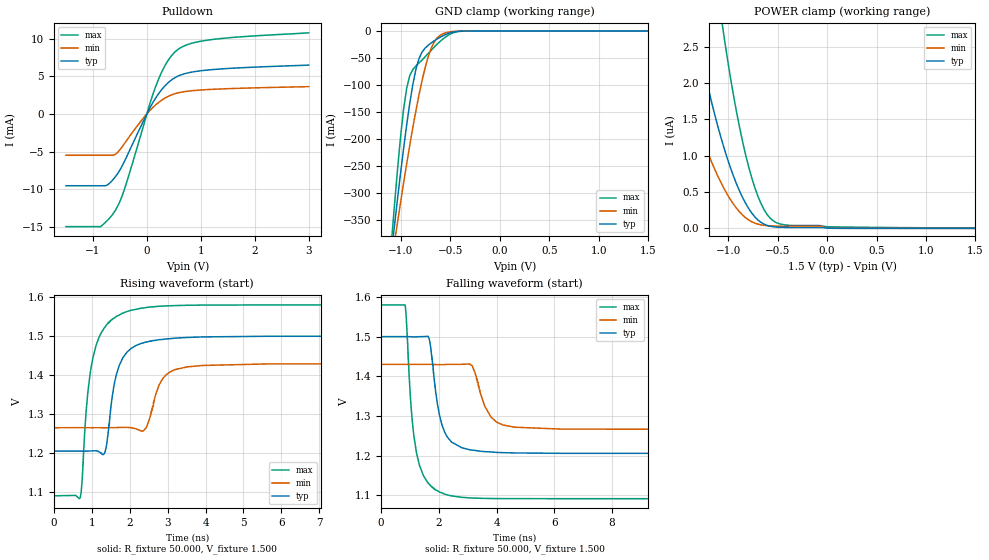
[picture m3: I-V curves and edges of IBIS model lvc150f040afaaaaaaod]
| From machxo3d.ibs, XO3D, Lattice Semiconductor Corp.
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|   Model lvc150f040afaaaaaaod
[Model] lvc150f040afaaaaaaod
Model_type I/O_open_drain
Polarity   Non-Inverting
Enable   Active-Low
Vinl =  0.375V
Vinh =  1.125V
Vmeas =  0.750V
Cref =  0.0F
Rref = 10.00k
Vref = 1.50V
C_comp   4.200pF   3.800pF   7.500pF
[Temperature Range]   25.000   0.105k   -40.000
[Voltage Range]   1.500V   1.430V   1.580V
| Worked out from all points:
|   slope of the pulldown table from 0 to 0.225 V, typ, clamps not added: 81.5 ohm
|   GND clamp passes 1 mA (typ) near -0.44 V on its own axis
|   rising waveform, R_fixture 50.000, V_fixture 1.500: 20-80 % time 357ps typ, 371ps min, 357ps max; typ from 1.21 V to 1.5 V
|   falling waveform, R_fixture 50.000, V_fixture 1.500: 20-80 % time 404ps typ, 495ps min, 361ps max; typ from 1.5 V to 1.21 V
[Pulldown]
|Voltage   I(typ)   I(min)   I(max)
-1.5V     -9.549mA   -5.496mA   -14.98mA
-856mV    -9.549mA   -5.496mA   -14.98mA
-718mV    -9.375mA   -5.496mA   -14.06mA
-580mV    -8.322mA   -5.363mA   -12.78mA
-396mV    -6.022mA   -3.748mA   -9.594mA
64mV      897.8uA    512.6uA    1.542mA
202mV     2.531mA    1.437mA    4.351mA
386mV     4.093mA    2.3mA      7.031mA
570mV     5.004mA    2.786mA    8.534mA
800mV     5.518mA    3.061mA    9.331mA
1.214V    5.895mA    3.272mA    9.897mA
3V        6.493mA    3.63mA     10.79mA
[GND_clamp]
|Voltage   I(typ)   I(min)   I(max)
-1.5V     -1.124A    -960.6mA   -1.411A
-1.097V   -411.6mA   -430.5mA   -392.9mA
-1.066V   -360.7mA   -392.1mA   -323mA
-1.035V   -311mA     -354.2mA   -256.8mA
-973mV    -216.9mA   -280.8mA   -144.3mA
-942mV    -173.5mA   -245.5mA   -105.7mA
-849mV    -71.07mA   -147.7mA   -64.62mA
-787mV    -39.18mA   -92.07mA   -53.7mA
-725mV    -26.42mA   -48.02mA   -41.6mA
-601mV    -11.16mA   -7.547mA   -18.74mA
-384mV    -237.5uA   -103.4uA   -356uA
1.5V      0A         0A         0A
[POWER_clamp]
|Voltage   I(typ)   I(min)   I(max)
-1.5V     4.017uA    2.297uA    8.486uA
-1.321V   2.676uA    1.475uA    5.815uA
-1.166V   1.719uA    902.9nA    3.892uA
-1.073V   1.242uA    625.4nA    2.92uA
-1.042V   1.099uA    544.2nA    2.626uA
-949mV    723.1nA    335.9nA    1.84uA
-856mV    425.6nA    184nA      1.196uA
-763mV    211.1nA    90.94nA    695.6nA
-670mV    83.03nA    48.42nA    343.1nA
-577mV    29.38nA    34.62nA    141nA
-422mV    12.83nA    29.5nA     47.28nA
1.5V      0A         0A         4.136nA
[Ramp]
| variable   typ   min   max
dV/dt_r   0.177/0.358n   98.704m/0.378n   0.293/0.357n
dV/dt_f   0.177/0.405n   98.705m/0.501n   0.293/0.354n
R_load = 50.000
[Rising Waveform]
R_fixture= 50.000
V_fixture= 1.500
V_fixture_min= 1.430
V_fixture_max= 1.580
|time   V(typ)   V(min)   V(max)
0s        1.205V     1.265V     1.091V
697ps     1.206V     1.266V     1.086V
953ps     1.206V     1.266V     1.401V
1.321ns   1.198V     1.265V     1.52V
1.65ns    1.402V     1.266V     1.551V
2.035ns   1.468V     1.266V     1.566V
2.422ns   1.485V     1.264V     1.573V
2.867ns   1.492V     1.391V     1.577V
3.518ns   1.497V     1.421V     1.579V
20ns      1.5V       1.43V      1.58V
[Falling Waveform]
R_fixture= 50.000
V_fixture= 1.500
V_fixture_min= 1.430
V_fixture_max= 1.580
|time   V(typ)   V(min)   V(max)
0s        1.5V       1.43V      1.58V
828ps     1.5V       1.43V      1.58V
1.044ns   1.5V       1.43V      1.317V
1.225ns   1.499V     1.43V      1.207V
1.666ns   1.495V     1.43V      1.128V
2.196ns   1.26V      1.429V     1.103V
3.151ns   1.214V     1.427V     1.093V
3.803ns   1.209V     1.297V     1.092V
4.628ns   1.207V     1.271V     1.091V
20ns      1.205V     1.265V     1.091V
